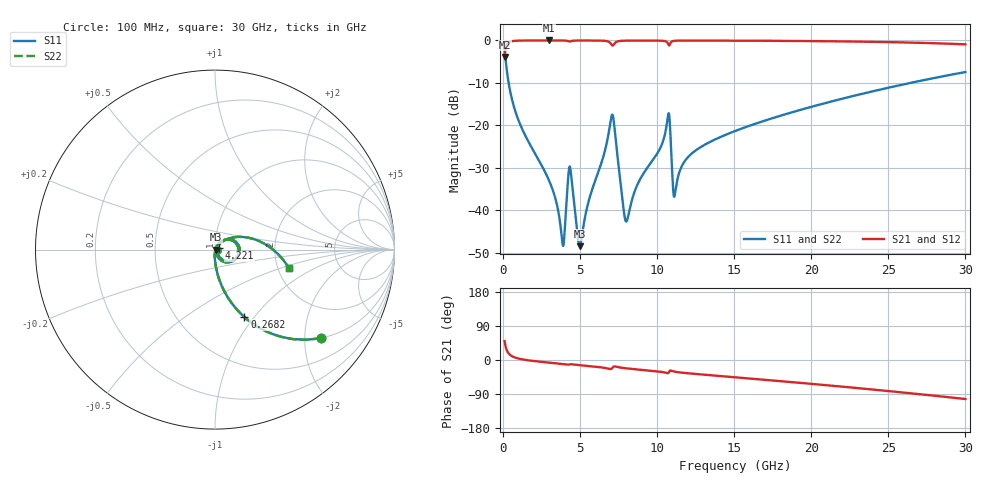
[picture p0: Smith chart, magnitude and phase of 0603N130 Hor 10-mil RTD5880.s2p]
# GHz S MA R 50
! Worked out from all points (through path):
!   3201 points, 100 MHz to 30 GHz, reference 50 ohm
!   highest |S21| = -0.02 dB at 2.959 GHz (marker M1); lowest = -3.9 dB at 100 MHz (marker M2)
!   group delay of S21, straight-line fit = 9.85 ps
!   lowest |S11| = -48.5 dB at 4.968 GHz (marker M3), VSWR 1.01, Z = 50.4 - j0.0491 ohm
!   |S11| at or under -10 dB: 360.5 MHz to 26.46 GHz (26.1 GHz wide, 195 % of centre)
!   |S22| runs from -48.5 to -2.3 dB; largest |S21 - S12| = 0
!   S11 on the Smith chart (normalised r, x): 100 MHz: 0.99, -2.40; 268.2 MHz: 0.99, -0.89; 4.221 GHz: 1.05, +0.01; 30 GHz: 2.30, -0.57
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0.1  0.7704 -39.9  0.6373 50.1  0.6373 50.1  0.7704 -39.9
0.2681875  0.4098 -66.5  0.9117 23.5  0.9117 23.5  0.4098 -66.5
1.006344  0.1138 -85.8  0.9926 3.8  0.9926 3.8  0.1138 -85.8
2.959188  0.02287 -92.8  0.9981 -6.8  0.9981 -6.8  0.02287 -92.8
3.865531  0.003952 -42.6  0.9966 -10.5  0.9966 -10.5  0.003952 -42.6
3.996344  0.005655 15.9  0.9949 -11.1  0.9949 -11.1  0.005655 15.9
4.220594  0.02362 17.1  0.9793 -12.3  0.9793 -12.3  0.02362 17.1
4.407469  0.02686 -47.6  0.9782 -11.2  0.9782 -11.2  0.02686 -47.6
4.968094  0.003761 -7.4  0.9962 -13.7  0.9962 -13.7  0.003761 -7.4
5.089563  0.004607 26.8  0.9964 -14.2  0.9964 -14.2  0.004607 26.8
7.05175  0.1304 5.2  0.8829 -22.8  0.8829 -22.8  0.1304 5.2
7.986125  0.007328 -9.1  0.9927 -22.0  0.9927 -22.0  0.007328 -9.1
8.780344  0.02111 52.5  0.9952 -25.2  0.9952 -25.2  0.02111 52.5
10.06978  0.04864 53.0  0.993 -30.2  0.993 -30.2  0.04864 53.0
10.72384  0.1355 7.8  0.8955 -34.5  0.8955 -34.5  0.1355 7.8
11.03219  0.01799 -36.6  0.982 -29.9  0.982 -29.9  0.01799 -36.6
11.15366  0.01556 16.2  0.9892 -31.0  0.9892 -31.0  0.01556 16.2
12.10672  0.04407 49.1  0.9947 -35.4  0.9947 -35.4  0.04407 49.1
15.05  0.08544 41.7  0.9921 -45.6  0.9921 -45.6  0.08544 41.7
20.03956  0.1656 25.3  0.9811 -63.0  0.9811 -63.0  0.1656 25.3
25.01978  0.2773 6.8  0.9545 -82.0  0.9545 -82.0  0.2773 6.8
30  0.4234 -13.9  0.8983 -102.9  0.8983 -102.9  0.4234 -13.9
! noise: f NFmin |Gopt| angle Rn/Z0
0.1  0.0003135  0.9239  0.4929  0.0009128
3.417  0.003815  0.8  9.418  0.003927
6.743  0.01686  0.9059  18.47  0.0383
10.06  0.0111  0.7999  27.38  0.01086
13.39  0.01062  0.7342  36.13  0.007231
16.7  0.01242  0.7215  44.63  0.007599
20.03  0.01454  0.7184  52.95  0.00824
23.35  0.01685  0.7201  61.03  0.008929
26.67  0.01941  0.7252  68.9  0.009657
30  0.0223  0.7333  76.56  0.01043
